(* Logix 5000 DataType export Banner_Black_Host_Out_Mirroring; software revision 33.00 *)

TYPE Banner_Black_Host_Out_Mirroring :
STRUCT
   Enable : SINT;   // 0=Disabled, 1=Enabled
   Port_Selection : SINT;   // 0=Port 1
   Channel_Selection : SINT;   // 0=Discrete 1, 1=Discrete 2
   Inversion : SINT;   // 0=Not Inverted, 1=Inverted
   Polarity : SINT;   // 0=NPN Output, 1=PNP Output
   Output_Type : SINT;   // 1=Output Open Collector, 2=Output Push Pull
END_STRUCT
END_TYPE
